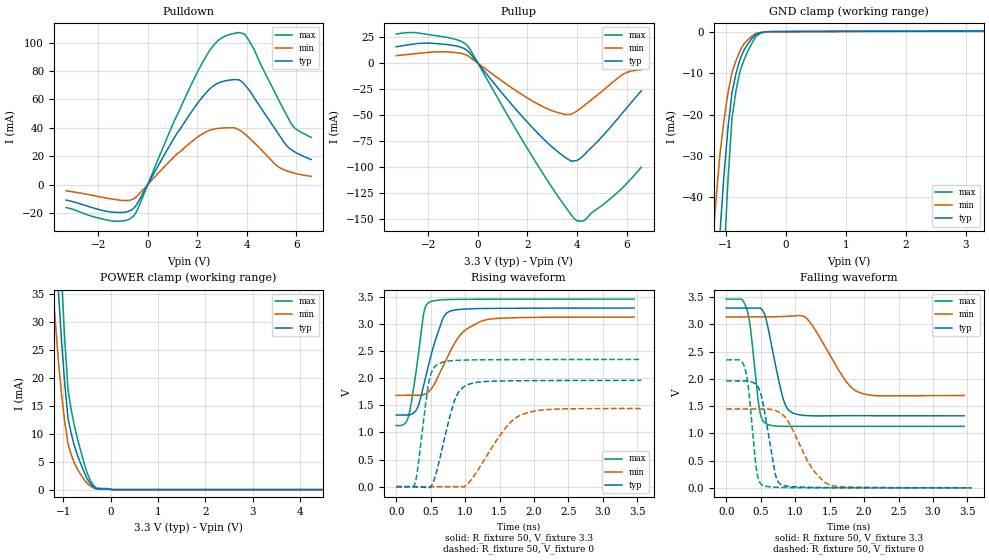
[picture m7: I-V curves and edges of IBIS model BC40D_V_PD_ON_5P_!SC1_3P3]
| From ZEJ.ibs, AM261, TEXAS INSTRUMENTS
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[Model]   BC40D_V_PD_ON_5P_!SC1_3P3
Model_type   I/O
Polarity   Non-Inverting
Enable   Active-Low
Vinl =  0.8V
Vinh =  2V
Cref =  15pF
Rref =  100.0000M
Vref =  0V
Vmeas =  1.65
C_comp   2.059994p   1.862014p   2.067327p
|[Input load] weak_pd_on
|[Output drive] fast
|[supplytol] 5
|[temp] ind
[Model Spec]
Vinl   0.8V   0.8V   0.8V
Vinh   2V   2V   2V
[Temperature Range]   25   125   -40
[Voltage Range]   3.3   3.135   3.465
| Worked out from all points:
|   slope of the pulldown table from 0 to 0.495 V, typ, clamps not added: 31.8 ohm
|   slope of the pullup table from 0 to 0.495 V, typ, clamps not added: 33.3 ohm
|   GND clamp passes 1 mA (typ) near -0.52 V on its own axis
|   POWER clamp passes 1 mA (typ) near -0.42 V on its own axis
|   rising waveform, R_fixture 50, V_fixture 3.3: 20-80 % time 251ps typ, 371ps min, 151ps max; typ from 1.32 V to 3.3 V
|   rising waveform, R_fixture 50, V_fixture 0: 20-80 % time 232ps typ, 456ps min, 140ps max; typ from 0 V to 1.96 V
|   falling waveform, R_fixture 50, V_fixture 3.3: 20-80 % time 196ps typ, 407ps min, 120ps max; typ from 3.3 V to 1.32 V
|   falling waveform, R_fixture 50, V_fixture 0: 20-80 % time 159ps typ, 359ps min, 107ps max; typ from 1.96 V to 0 V
| Nom Voltages:
|   VDD=1.1, VDDS=3.3, VDDS18=1.8, ESD_BIASFET=0, VSS=0, VSSS=0
| Min Voltages:
|   VDD=1.045, VDDS=3.135, VDDS18=1.71, ESD_BIASFET=0, VSS=0, VSSS=0
| Max Voltages:
|   VDD=1.16, VDDS=3.465, VDDS18=1.89, ESD_BIASFET=0, VSS=0, VSSS=0
[POWER_clamp]
|   voltage   I(typ)   I(min)   I(max)
-3.3V     446.9mA    437.1mA    604mA
-1.233V   56.59mA    37.52mA    80.37mA
-1.167V   45.68mA    29.91mA    65.17mA
-1.1V     35.14mA    22.67mA    50.36mA
-1.033V   26.13mA    16.78mA    37.31mA
-966.7mV  18.67mA    11.95mA    26.46mA
-900mV    12.76mA    8.173mA    17.82mA
-833.3mV  10.07mA    6.293mA    14.34mA
-566.7mV  3.276mA    1.91mA     4.968mA
-366.7mV  519.9uA    314uA      774.5uA
33.33mV   0A         0A         0A
6.6V      0A         0A         0A
[Pulldown]
|   voltage   I(typ)   I(min)   I(max)
-3.3V     -10.92mA   -4.469mA   -16.24mA
-1.4V     -19.52mA   -10.37mA   -25.81mA
-600mV    -17.22mA   -10.34mA   -22.6mA
-400mV    -12.67mA   -7.623mA   -17.05mA
1.2V      36.7mA     21.92mA    49.35mA
2.1V      59.3mA     34.49mA    82.4mA
2.7V      70.09mA    39.15mA    99.03mA
3.3V      73.56mA    39.95mA    105.7mA
3.9V      70.66mA    35.84mA    106mA
5.2V      37.64mA    13.39mA    62.46mA
5.8V      24.43mA    8.578mA    42.66mA
6.6V      17.6mA     5.765mA    33.17mA
[Pullup]
|   voltage   I(typ)   I(min)   I(max)
-3.3V     15.77mA    7.22mA     28.03mA
-1.9V     19.23mA    10.53mA    27.2mA
-900mV    16.69mA    10.25mA    22.94mA
-400mV    11.53mA    6.969mA    16.15mA
1.4V      -40.96mA   -24.37mA   -58.54mA
2.6V      -72.01mA   -41.71mA   -105.6mA
3.5V      -90.51mA   -49.41mA   -137.6mA
3.8V      -94.64mA   -48.83mA   -147.5mA
4V        -93.88mA   -46.2mA    -152.2mA
4.3V      -88.33mA   -40.72mA   -151.7mA
5.9V      -46.29mA   -10.2mA    -118.8mA
6.6V      -26.71mA   -6.269mA   -100.4mA
[GND_clamp]
|   voltage   I(typ)   I(min)   I(max)
-3.3V     -787.2mA   -627.7mA   -1.235A
-1.233V   -85.66mA   -52.14mA   -138.8mA
-1.167V   -66.47mA   -40.37mA   -107.7mA
-1.1V     -48.25mA   -29.37mA   -77.98mA
-1.033V   -34.28mA   -21.19mA   -54.56mA
-966.7mV  -23.07mA   -14.67mA   -35.51mA
-900mV    -14.62mA   -9.792mA   -20.84mA
-833.3mV  -10.07mA   -6.939mA   -14.17mA
-700mV    -4.435mA   -2.94mA    -6.836mA
-500mV    -641.2uA   -454.9uA   -1.12mA
-300mV    -31.62uA   -32.88uA   -44.11uA
3.3V      108.6uA    60.68uA    188uA
[Ramp]
| variable   typ   min   max
dV/dt_f  1.1955351/0.19759568n 0.88985276/0.4200075n  1.4066392/0.12028585n
dV/dt_r  1.1906978/0.23429938n 0.88860778/0.46756332n  1.4192328/0.14138141n
R_load = 50
[Rising Waveform]
R_fixture = 50
V_fixture = 3.3
V_fixture_min = 3.135
V_fixture_max = 3.465
|   time   V(typ)   V(min)   V(max)
0s        1.321V     1.685V     1.128V
178.2ps   1.322V     1.685V     1.295V
301.2ps   1.435V     1.685V     2.241V
400ps     1.877V     1.699V     3.202V
481.7ps   2.307V     1.764V     3.404V
656.6ps   3.033V     2.161V     3.449V
724.7ps   3.194V     2.347V     3.453V
946.4ps   3.274V     2.825V     3.458V
1.232ns   3.288V     3.053V     3.46V
3.453ns   3.297V     3.129V     3.462V
[Rising Waveform]
R_fixture = 50
V_fixture = 0
V_fixture_min = 0
V_fixture_max = 0
|   time   V(typ)   V(min)   V(max)
0s        0V         0V         0V
272.8ps   -6.681mV   0V         57.86mV
474.8ps   -20.71mV   0V         1.934V
537.3ps   78.74mV    0V         2.176V
615.7ps   426mV      0V         2.269V
850ps     1.601V     0V         2.33V
1.039ns   1.882V     56.1mV     2.338V
1.571ns   1.952V     1.06V      2.345V
1.827ns   1.956V     1.332V     2.346V
3.559ns   1.962V     1.442V     2.348V
[Falling Waveform]
R_fixture = 50
V_fixture = 3.3
V_fixture_min = 3.135
V_fixture_max = 3.465
|   time   V(typ)   V(min)   V(max)
0s        3.297V     3.134V     3.461V
297.1ps   3.297V     3.134V     3.274V
347.5ps   3.297V     3.134V     2.957V
481.9ps   3.297V     3.134V     1.432V
580.8ps   3.074V     3.135V     1.176V
820.1ps   1.656V     3.142V     1.128V
962.4ps   1.375V     3.152V     1.128V
1.188ns   1.324V     3.078V     1.129V
1.913ns   1.324V     1.758V     1.127V
3.453ns   1.321V     1.694V     1.127V
[Falling Waveform]
R_fixture = 50
V_fixture = 0
V_fixture_min = 0
V_fixture_max = 0
|   time   V(typ)   V(min)   V(max)
0s        1.961V     1.446V     2.348V
273.4ps   1.961V     1.446V     2.176V
323.8ps   1.957V     1.446V     1.804V
436.6ps   1.887V     1.446V     343mV
524.2ps   1.599V     1.446V     49.34mV
710.3ps   256.3mV    1.419V     11.45mV
807.8ps   53.46mV    1.353V     6.57mV
1.236ns   9.417mV    373.9mV    0V
1.49ns    5.81mV     57.56mV    0V
3.559ns   0V         2.809mV    0V
